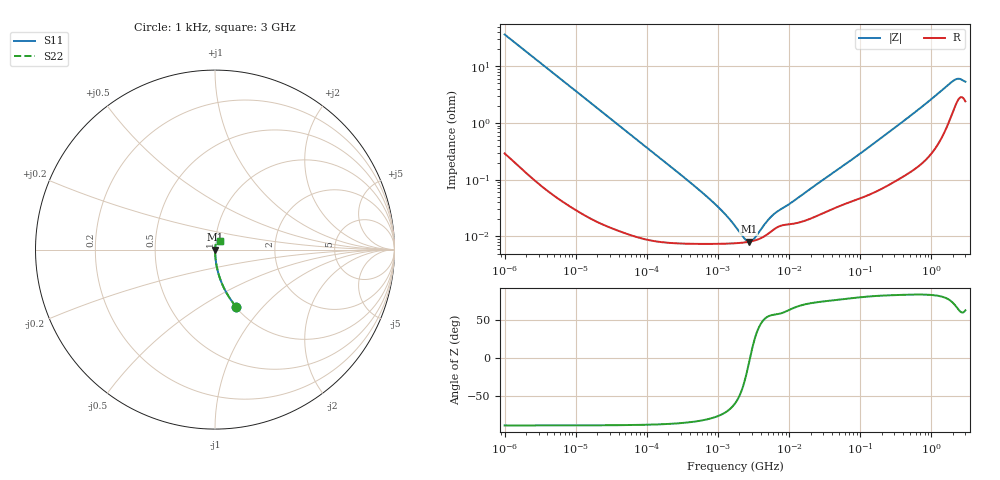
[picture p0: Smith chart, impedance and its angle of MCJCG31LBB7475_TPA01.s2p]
! MCJCG31LBB7475_TPA01  S-PARAMETER MODEL  ( Standard Model )
! Model Generated by TAIYO YUDEN Corporation (http://www.ty-top.com)
! Version 1.0
! TAIYO YUDEN Control No. 220601
! Copyright(c) 2015 TAIYO YUDEN CO.,LTD. All Rights Reserved.
! Product Description (link to TY-COMPAS)
! https://ds.yuden.co.jp/TYCOMPAS/or/detail?pn=MCJCG31LBB7475KTPA01&u=M
! Products Name : Multilayer Ceramic Capacitors
! Characteristics :
!  Capacitance : 4.7 [uF] , Rated Voltage : 35 [V] , TCC : X7R
!  Case Size : 3.2 x 1.6 / 0.126 x 0.063 [mm/inch] , Thickness : 1.6 / 0.063 [mm/inch]
!  (Conditions: Temperature = 25 [degC] , DC Bias Voltage = 0 [V])
! External Node Assignments :
!  1  o---| |---o  2
! GND o---------o GND
! Frequency Range : 1kHz  -  3GHz  [ 401 STEP ]
# MHZ S RI R 50
! Freq[MHz].  S11 Real  S11 Imag  S21 Real  S21 Imag  S12 Real  S12 Imag  S22 Real  S22 Imag
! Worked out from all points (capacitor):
!   401 points, 1 kHz to 3 GHz, reference 50 ohm
!   read as one part in series: C = 4.38 uF near 1.077 kHz
!   lowest |Z| = 8.11 mohm at 2.709 MHz (marker M1)
!   series resonance near 2.817 MHz, so ESL is about 730 pH
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0.001  0.1181 -0.3187  0.8819 0.3187  0.8819 0.3187  0.1181 -0.3187
0.001685  0.0458 -0.2054  0.9542 0.2054  0.9542 0.2054  0.0458 -0.2054
0.00306  0.0148 -0.1172  0.9852 0.1172  0.9852 0.1172  0.0148 -0.1172
0.005768  0.00444 -0.063  0.9956 0.063  0.9956 0.063  0.00444 -0.063
0.01216  0.00116 -0.0301  0.9988 0.0301  0.9988 0.0301  0.00116 -0.0301
0.147855  8.66e-05 -0.00249  0.9999 0.00249  0.9999 0.00249  8.66e-05 -0.00249
0.791611  7.41e-05 -0.000431  0.9999 0.000431  0.9999 0.000431  7.41e-05 -0.000431
1.238299  7.45e-05 -0.000242  0.9999 0.000242  0.9999 0.000242  7.45e-05 -0.000242
1.732051  7.58e-05 -0.000133  0.9999 0.000133  0.9999 0.000133  7.58e-05 -0.000133
2.166294  7.75e-05 -7.02e-05  0.9999 7.02e-05  0.9999 7.02e-05  7.75e-05 -7.02e-05
2.334012  7.83e-05 -5.01e-05  0.9999 5.01e-05  0.9999 5.01e-05  7.83e-05 -5.01e-05
2.709407  8.05e-05 -1.03e-05  0.9999 1.03e-05  0.9999 1.03e-05  8.05e-05 -1.03e-05
3.388684  8.6e-05 4.94e-05  0.9999 -4.94e-05  0.9999 -4.94e-05  8.6e-05 4.94e-05
4.919932  0.000109 0.000153  0.9999 -0.000153  0.9999 -0.000153  0.000109 0.000153
6.153411  0.000134 0.000211  0.9999 -0.000211  0.9999 -0.000211  0.000134 0.000211
21.06097  0.000212 0.000697  0.9998 -0.000697  0.9998 -0.000697  0.000212 0.000697
83.67817  0.000439 0.00242  0.9996 -0.00242  0.9996 -0.00242  0.000439 0.00242
256.0921  0.000865 0.00693  0.9991 -0.00693  0.9991 -0.00693  0.000865 0.00693
700.8126  0.00217 0.0182  0.9978 -0.0182  0.9978 -0.0182  0.00217 0.0182
1990.675  0.0178 0.0505  0.9822 -0.0505  0.9822 -0.0505  0.0178 0.0505
2398.636  0.0281 0.0514  0.9719 -0.0514  0.9719 -0.0514  0.0281 0.0514
3000  0.0256 0.0455  0.9744 -0.0455  0.9744 -0.0455  0.0256 0.0455
